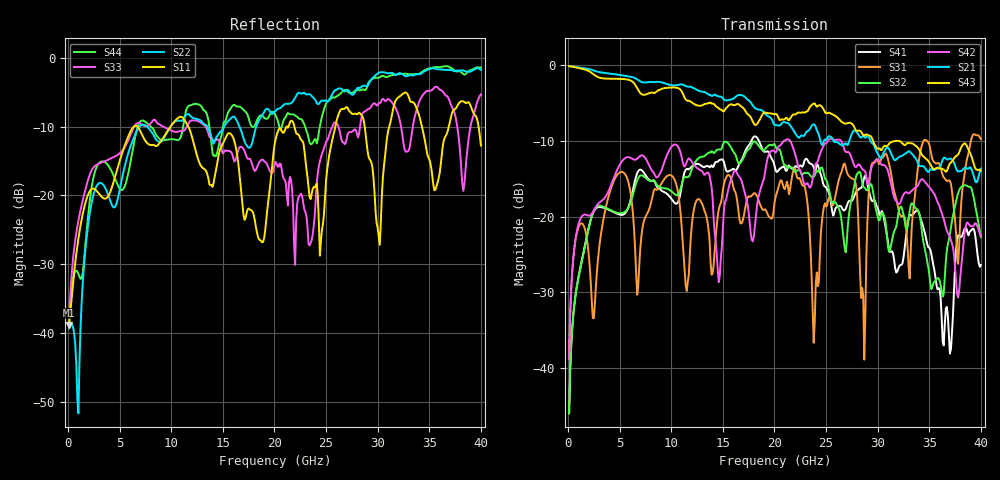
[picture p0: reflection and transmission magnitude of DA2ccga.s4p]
! ADC12DJ3200QML-SP
! 196-pin NWE package
! CCGA Ceramic Package with columns (ceramic column grid array)
! Texas Instruments 4/21/2021
! Single-ended  S-parameters
! PORT#  PORT_NAME  NET_NAME
! PORT1:  DAxN.DIEBUMP DAxN
! PORT2:  DAxN.BGA  DAxN
! PORT3:  DAxP.DIEBUMP DAxP
! PORT4:  DAxP.BGA  DAxP
! Touchstone Ver. 1.0
! Number of ports is 4
# Hz	S	MA	R	50.000000
! SCATTERING PARAMETERS  :
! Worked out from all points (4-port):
!   400 points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, 100 MHz to 40 GHz, reference 50 ohm
!   strongest paths, dB at 100 MHz, 10.1 GHz, 20.1 GHz, 30.1 GHz, 40 GHz:
!     S43: -0.1, -2.9, -6.4, -11.0, -13.9
!     S21: -0.1, -2.6, -7.9, -11.9, -13.7
!     S42: -38.8, -10.6, -11.5, -12.5, -22.6
!     S32: -46.0, -16.8, -10.7, -20.5, -22.7
!     S31: -38.8, -14.7, -17.5, -13.0, -9.7
!     S41: -46.0, -17.8, -13.8, -19.3, -26.4
!   lowest |S11| = -38.8 dB at 100 MHz (marker M1), VSWR 1.02, Z = 51.1 + j0.184 ohm
!   |S11| at or under -10 dB: start of sweep to 6.367 GHz; 11.64 GHz to 21.18 GHz (9.541 GHz wide, 58.2 % of centre); 21.93 GHz to 25.9 GHz (3.964 GHz wide, 16.6 % of centre)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
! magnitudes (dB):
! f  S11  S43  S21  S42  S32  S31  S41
! 100 MHz  -38.8  -0.1  -0.1  -38.8  -46.0  -38.8  -46.0
! 6.9 GHz  -10.4  -3.5  -2.0  -12.1  -14.7  -26.4  -13.8
! 23.8 GHz  -18.8  -5.0  -7.8  -14.3  -14.7  -36.7  -13.5
! 26.8 GHz  -7.4  -7.7  -10.3  -11.2  -24.1  -13.0  -19.1
! 28.7 GHz  -9.6  -9.3  -9.4  -13.9  -16.1  -38.9  -14.8
! 29.5 GHz  -16.1  -9.8  -10.3  -13.2  -16.3  -12.9  -18.0
! 40 GHz  -12.7  -13.9  -13.7  -22.6  -22.7  -9.7  -26.4
